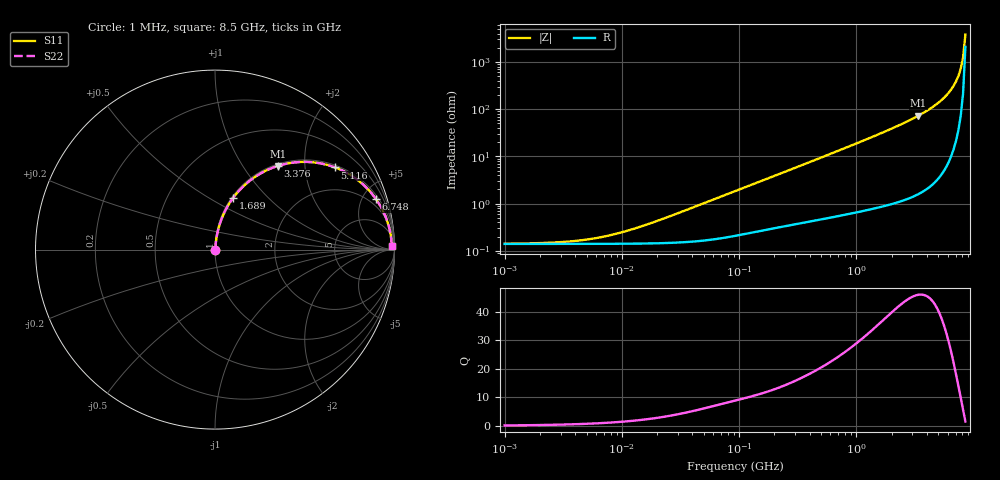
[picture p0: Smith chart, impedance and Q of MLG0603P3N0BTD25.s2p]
! S-Parameter Data Generated by TDK Corporation
! Copyright(C) 2025 TDK Corporation.
! All Rights Reserved.
! TDK P/N: MLG0603P3N0BTD25 (SMD / SMT Inductor (Coil))
! Property: L=3nH at 500MHz
! Size(LxWxT): 0.6x0.3x0.3mm
! Model Type: s2p (Touchstone File Format Version 1.0)
! Frequency: DC=Yes Start=1MHz Stop=8500MHz 198points Log-sweep
! Model Generated on Feb. 6, 2025
! Terms and conditions regarding TDK Simulation Models:
! 1)This simulation model is being provided solely for informational
!  purposes. Please refer to the specifications of the products in
!  terms of detailed characteristics of such products.
! 2)In no event shall TDK Corporation of any of its subsidiaries be
!  liable for any loss or damage arising, directly or indirectly,
!  from any information contained in this simulation model, including,
!  but not limited to loss or damages arising from any inaccuracies,
!  omissions or errors in connection with such information.
! 3)Any and all copyrights on this simulation model are owned by
!  TDK Corporation.  Duplication or redistribution of this simulation
!  model without prior written permission from TDK Corporation
!  is prohibited.
! 4)This simulation model is subject to any modification or change
!  without any prior notice.
! 5)Neither TDK Corporation nor any of its subsidiaries shall make any
!  warranty, express or implied, including but not limited to the
!  correctness, implied warranties of merchantability and fitness for
!  a particular purpose with respect to this simulation models.
! 6)The use of this simulation model shall be deemed to have consented
!  to the terms and conditions hereof.
! Port Assignments:
!  1 ---@@@--- 2
! Applicable Conditions:
!  Temperature = 25 degC
!  DC Bias Current = 0 A
!  Small Signal Operation
# Hz S MA R 50
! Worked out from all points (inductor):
!   197 points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, 1 MHz to 8.5 GHz, reference 50 ohm
!   read as one part in series: L = 3.22 nH near 22.04 MHz
!   highest Q = 45.9 at 3.376 GHz (marker M1), where L = 3.43 nH
!   S11 on the Smith chart (normalised r, x): 1 MHz: 1.00, +0.00; 1.689 GHz: 1.02, +0.65; 3.376 GHz: 1.03, +1.46; 5.116 GHz: 1.07, +2.87; 6.748 GHz: 1.28, +6.27; 8.5 GHz: 43, +64
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1000000  0.001413 8.2  0.9986 -0.0  0.9986 -0.0  0.001413 8.2
2517452  0.001489 20.0  0.9986 -0.0  0.9986 -0.0  0.001489 20.0
4587603  0.001681 33.5  0.9986 -0.1  0.9986 -0.1  0.001681 33.5
6636977  0.001943 43.7  0.9986 -0.1  0.9986 -0.1  0.001943 43.7
9168677  0.00233 52.7  0.9986 -0.1  0.9986 -0.1  0.00233 52.7
2.10461e7  0.004495 71.0  0.9985 -0.2  0.9985 -0.2  0.004495 71.0
9.219544e7  0.01836 82.5  0.9978 -1.0  0.9978 -1.0  0.01836 82.5
4.229561e8  0.07949 82.4  0.9926 -4.6  0.9926 -4.6  0.07949 82.4
8.852465e8  0.1631 78.5  0.9806 -9.4  0.9806 -9.4  0.1631 78.5
1.689417e9  0.3053 70.7  0.944 -17.8  0.944 -17.8  0.3053 70.7
1.940355e9  0.3487 68.1  0.9284 -20.4  0.9284 -20.4  0.3487 68.1
2.559585e9  0.4531 61.7  0.8811 -26.9  0.8811 -26.9  0.4531 61.7
3.37643e9  0.5828 53.1  0.8 -35.6  0.8 -35.6  0.5828 53.1
4.253027e9  0.7076 43.7  0.6909 -45.0  0.6909 -45.0  0.7076 43.7
5.115526e9  0.8108 34.4  0.5651 -54.2  0.5651 -54.2  0.8108 34.4
5.87536e9  0.8824 26.3  0.4438 -61.9  0.4438 -61.9  0.8824 26.3
6.748056e9  0.9406 17.4  0.2996 -70.0  0.2996 -70.0  0.9406 17.4
7.066863e9  0.9555 14.3  0.247 -72.6  0.247 -72.6  0.9555 14.3
7.400733e9  0.9677 11.1  0.1926 -74.9  0.1926 -74.9  0.9677 11.1
7.750377e9  0.9769 7.8  0.1369 -76.4  0.1369 -76.4  0.9769 7.8
8.116539e9  0.983 4.5  0.0804 -75.5  0.0804 -75.5  0.983 4.5
8.5e9  0.9857 1.2  0.02575 -55.6  0.02575 -55.6  0.9857 1.2
